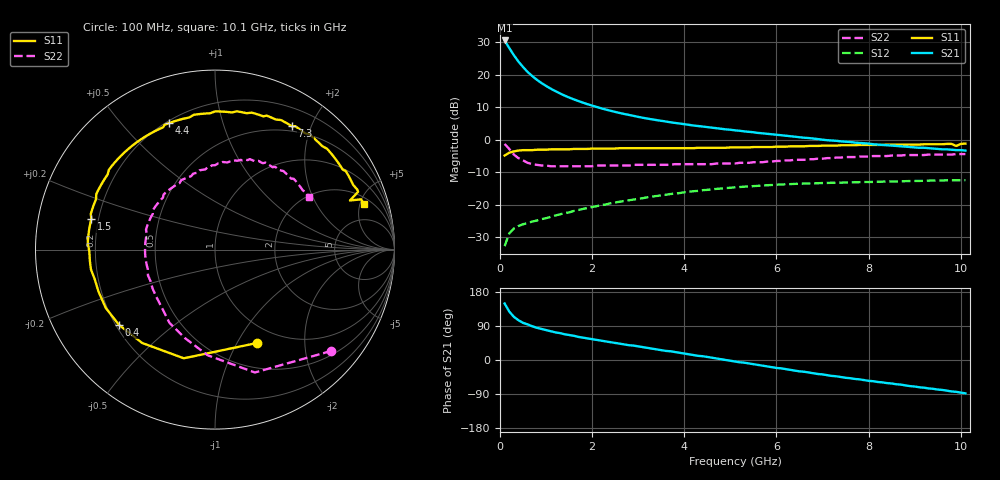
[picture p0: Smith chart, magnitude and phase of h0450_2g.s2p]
!HBFP-0450
!S and NOISE PARAMETERS at Vce=2V  Ic=35mA.  LAST UPDATED  09-04-98
# GHZ S MA R  50
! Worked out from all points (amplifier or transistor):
!   101 points, 100 MHz to 10.1 GHz, reference 50 ohm
!   highest |S21| = 30.5 dB at 100 MHz (marker M1)
!   |S21| within 3 dB of that: start of sweep to 231.3 MHz
!   unconditionally stable (mu >= 1): 2.221 GHz to end of sweep
!   at 1.7 GHz: K = 0.93, MSG = 16.8 dB, |S12| = -21.6 dB
!   at 5.1 GHz: K = 1.08, MAG = 7.0 dB, |S12| = -14.7 dB
!   at 10.1 GHz: K = 1.04, MAG = 3.3 dB, |S12| = -12.5 dB
!   lowest NFmin = 1.55 dB at 1.8 GHz
!   S11 on the Smith chart (normalised r, x): 100 MHz: 0.78, -1.21; 400 MHz: 0.21, -0.33; 1.5 GHz: 0.17, +0.12; 4.4 GHz: 0.21, +0.68; 7.3 GHz: 0.43, +1.72; 10.1 GHz: 2.62, +5.47
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0.1  0.57 -66.0  33.56 149.0  0.023 64.0  0.86 -41.0
0.2  0.63 -106.0  25.74 128.0  0.036 49.0  0.72 -72.0
0.3  0.66 -128.0  19.93 114.0  0.043 41.0  0.59 -94.0
0.4  0.68 -142.0  15.91 105.0  0.047 37.0  0.52 -109.0
0.5  0.69 -152.0  13.1 98.0  0.05 35.0  0.48 -122.0
0.6  0.69 -160.0  11 94.0  0.052 35.0  0.44 -132.0
0.7  0.69 -166.0  9.5 89.0  0.055 35.0  0.42 -141.0
0.8  0.7 -171.0  8.34 85.0  0.057 35.0  0.41 -148.0
0.9  0.7 -175.0  7.43 82.0  0.06 35.0  0.4 -154.0
1.1  0.71 177.0  6.09 76.0  0.065 35.0  0.39 -164.0
1.3  0.71 171.0  5.15 71.0  0.071 36.0  0.39 -172.0
1.5  0.71 166.0  4.45 66.0  0.076 35.0  0.39 -179.0
1.8  0.72 159.0  3.71 59.0  0.086 34.0  0.39 172.0
2.2  0.73 151.0  3.03 51.0  0.098 32.0  0.4 162.0
2.5  0.73 145.0  2.67 45.0  0.108 30.0  0.4 156.0
3.5  0.74 126.0  1.95 26.0  0.139 21.0  0.41 138.0
4.4  0.75 110.0  1.59 10.0  0.167 10.0  0.42 122.0
5.1  0.76 97.0  1.39 -4.0  0.185 0.0  0.43 108.0
6.8  0.8 67.0  1.04 -35.0  0.213 -24.0  0.5 79.0
7.3  0.81 58.0  0.96 -43.0  0.218 -31.0  0.53 71.0
8.5  0.84 41.0  0.81 -62.0  0.228 -47.0  0.57 54.0
10.1  0.87 17.0  0.68 -88.0  0.238 -69.0  0.6 29.0
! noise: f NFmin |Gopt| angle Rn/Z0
1.8  1.55  0.55  -157  0.08
2  1.6  0.55  -155  0.08
2.5  1.72  0.58  -145  0.12
3.5  1.96  0.63  -127  0.25
4  2.09  0.66  -116  0.38
4.5  2.18  0.68  -108  0.52
5.5  2.45  0.72  -88  0.98
6  2.57  0.73  -80  1.21
7  2.83  0.76  -61  2.03
9  3.31  0.82  -31  3.75
